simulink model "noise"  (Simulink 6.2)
settings: Solver=ode4  StartTime=0.0  StopTime=20  FixedStep=.01  RelTol=1e-3

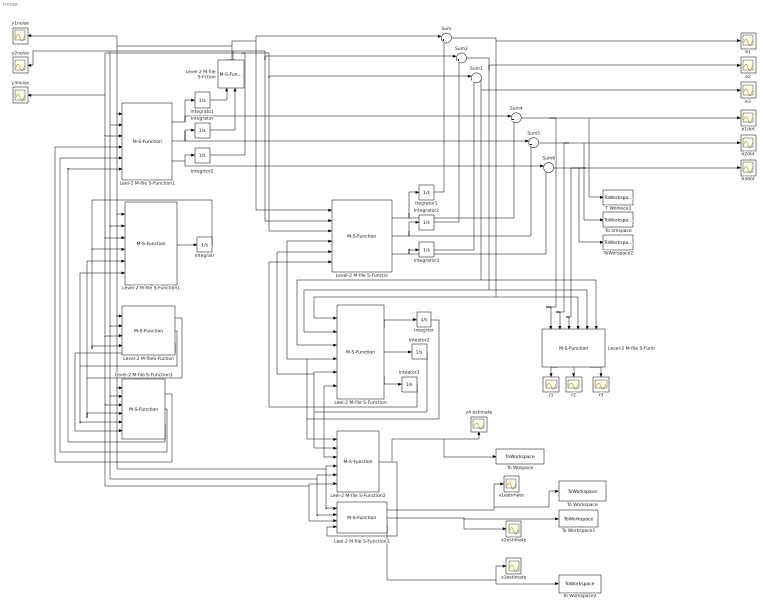
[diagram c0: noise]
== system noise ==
  Inteator2 : Integrator  InitialCondition=1
  Inteator3 : Integrator  InitialCondition=1
  Integrato1 : Integrator  InitialCondition=.769
  Integrator : Integrator  InitialCondition=1.15
  Integrator2 : Integrator  InitialCondition=1.15
  Integrator3 : Integrator  InitialCondition=1.92
  Integratr : Integrator  InitialCondition=1.92
  Integrtor : Integrator  InitialCondition=1
  Integrtor2 : Integrator  InitialCondition=1.92
  Itegrator1 : Integrator  InitialCondition=.769
  Leel-2 M-file S-Function : M-S-Function  MFile=f_123estimate
  Leel-2 M-file S-Function1 : M-S-Function  MFile=y_dynamics123
  Leel-2 M-file S-Function2 : M-S-Function  MFile=y_4estimate
  Leel-2 M-file S-Function3 : M-S-Function  MFile=x_123estimate
  Level-2 M-file S-Fction : M-S-Function  Orientation=up  MFile=y_12noise
  Level-2 M-file S-Functio : M-S-Function  MFile=y_dynamics123estimate
  Level-2 M-file S-Function1 : M-S-Function  MFile=y_dynamics4
  Level-2 M-file S-Function3 : M-S-Function  MFile=f_123
  Level-2 M-file S-Funti : M-S-Function  Orientation=down  MFile=r_123
  Level-2 M-fileS-Fuction : M-S-Function  MFile=y_567
  Sum{,1..2,4..6} (6 alike) : Sum  Inputs=|+-
  T Worksce1 : ToWorkspace  VariableName=e1dot_noise  SampleTime=-1  SaveFormat=Array
  To Workspace : ToWorkspace  VariableName=x1estimate_noise  SampleTime=-1  SaveFormat=Array
  To Workspace1 : ToWorkspace  VariableName=x2estimate_noise  SampleTime=-1  SaveFormat=Array
  To Workspace2 : ToWorkspace  VariableName=x3estimate_noise  SampleTime=-1  SaveFormat=Array
  To Wospace : ToWorkspace  VariableName=y4estimate_noise  SampleTime=-1  SaveFormat=Array
  To orkspace : ToWorkspace  VariableName=e2dot_noise  SampleTime=-1  SaveFormat=Array
  ToWorspace2 : ToWorkspace  VariableName=e3dot_noise  SampleTime=-1  SaveFormat=Array
  e1 : Scope
  e1dot : Scope
  e2 : Scope
  e2dot : Scope
  e3 : Scope
  e3dot : Scope
  r1 : Scope
  r2 : Scope
  r3 : Scope
  x1estimate : Scope
  x2estimate : Scope
  x3estimate : Scope
  y1noise : Scope
  y2noise : Scope
  y3noise : Scope
  y4 estimate : Scope
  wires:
  Leel-2 M-file S-Function1/1 -> Integrato1/1, Sum4/1
  Leel-2 M-file S-Function1/2 -> Sum5/1, Integrator/1
  Leel-2 M-file S-Function1/3 -> Integrtor2/1, Sum6/1
  Level-2 M-file S-Functio/1 -> Itegrator1/1, Sum4/2
  Level-2 M-file S-Functio/2 -> Integrator2/1, Sum5/2
  Level-2 M-file S-Functio/3 -> Integrator3/1, Sum6/2
  Itegrator1/1 -> Sum/2
  Integrator2/1 -> Sum2/2
  Integrator3/1 -> Sum1/2
  Sum1/1 -> e3/1, Leel-2 M-file S-Function/3, Level-2 M-file S-Funti/6
  Sum2/1 -> e2/1, Leel-2 M-file S-Function/2, Level-2 M-file S-Funti/5
  Sum/1 -> e1/1, Leel-2 M-file S-Function/1, Level-2 M-file S-Funti/4
  Leel-2 M-file S-Function/1 -> Integrtor/1
  Leel-2 M-file S-Function/2 -> Inteator2/1
  Leel-2 M-file S-Function/3 -> Inteator3/1
  Inteator3/1 -> Leel-2 M-file S-Function/6, Level-2 M-file S-Functio/6, Leel-2 M-file S-Function2/3
  Inteator2/1 -> Leel-2 M-file S-Function/5, Level-2 M-file S-Functio/5, Leel-2 M-file S-Function2/2
  Integrtor/1 -> Leel-2 M-file S-Function/4, Level-2 M-file S-Functio/4, Leel-2 M-file S-Function2/1
  Sum4/1 -> Level-2 M-file S-Funti/1, e1dot/1, T Worksce1/1
  Sum5/1 -> Level-2 M-file S-Funti/2, e2dot/1, To orkspace/1
  Sum6/1 -> e3dot/1, Level-2 M-file S-Funti/3, ToWorspace2/1
  Level-2 M-file S-Funti/1 -> r1/1
  Level-2 M-file S-Funti/2 -> r2/1
  Level-2 M-file S-Funti/3 -> r3/1
  Level-2 M-file S-Function1/1 -> Integratr/1
  Integratr/1 -> Level-2 M-file S-Function1/4, Level-2 M-fileS-Fuction/4
  Level-2 M-fileS-Fuction/3 -> Level-2 M-file S-Function3/6
  Level-2 M-fileS-Fuction/2 -> Level-2 M-file S-Function3/5, Level-2 M-file S-Function1/6
  Level-2 M-fileS-Fuction/1 -> Level-2 M-file S-Function3/4, Level-2 M-file S-Function1/5
  Level-2 M-file S-Function3/3 -> Leel-2 M-file S-Function1/6
  Level-2 M-file S-Function3/2 -> Leel-2 M-file S-Function1/5
  Level-2 M-file S-Function3/1 -> Leel-2 M-file S-Function1/4
  Leel-2 M-file S-Function2/1 -> Leel-2 M-file S-Function3/4, y4 estimate/1, To Wospace/1
  Leel-2 M-file S-Function3/1 -> x1estimate/1, To Workspace/1
  Leel-2 M-file S-Function3/2 -> x2estimate/1, To Workspace1/1
  Leel-2 M-file S-Function3/3 -> x3estimate/1, To Workspace2/1
  Level-2 M-file S-Fction/2 -> Leel-2 M-file S-Function1/2, Level-2 M-file S-Function1/2, Level-2 M-fileS-Fuction/2, Level-2 M-file S-Function3/2, Leel-2 M-file S-Function2/5, Leel-2 M-file S-Function3/2, y2noise/1, Sum2/1, Level-2 M-file S-Functio/2
  Integrator/1 -> Level-2 M-file S-Fction/2
  Integrtor2/1 -> Leel-2 M-file S-Function1/3, Level-2 M-file S-Function1/3, Level-2 M-fileS-Fuction/3, Level-2 M-file S-Function3/3, Leel-2 M-file S-Function2/6, Leel-2 M-file S-Function3/3, y3noise/1, Sum1/1, Level-2 M-file S-Functio/3
  Level-2 M-file S-Fction/1 -> Leel-2 M-file S-Function1/1, Level-2 M-file S-Function1/1, Level-2 M-fileS-Fuction/1, Level-2 M-file S-Function3/1, Leel-2 M-file S-Function2/4, Leel-2 M-file S-Function3/1, y1noise/1, Sum/1, Level-2 M-file S-Functio/1
  Integrato1/1 -> Level-2 M-file S-Fction/1
